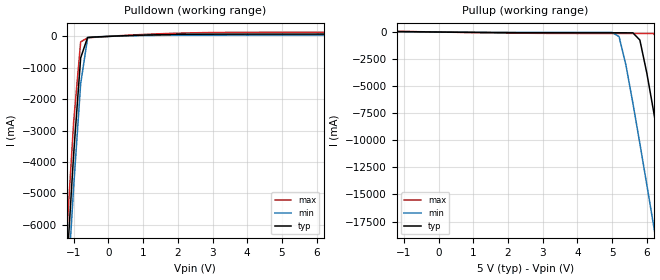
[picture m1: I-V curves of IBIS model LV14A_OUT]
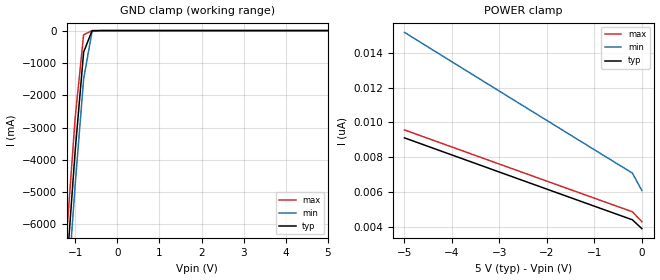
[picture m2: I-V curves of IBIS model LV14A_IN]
|   TEXAS INSTRUMENTS INCORPORATED
|   Advanced Bus Interface Group
|   IBIS Model of LV14A (Vcc=5V)
|   CMOS Hex Schmitt-Trigger Inverter
|   SOIC 14-pin (D) Package
[IBIS Ver]   1.1
[File Name]   lv14a_5.ibs
[File Rev]   2.0
[Date]   9/6/97
[Source]   File originated at Texas Instruments, Inc.
[Notes]   The following is an IBIS list for the LV14A.
|   - All test data contained in this file are derived from
|   hspice(tm) simulations.
|   - File created by Teruo Ishii, SLL Applications.
[Disclaimer] Property of Texas Instruments Incorporated.  Unauthorized
   reproduction and/or distribution is strictly prohibited.
   This product is protected under copyright law.
   Created 1997, (C) Copyright 1997, Texas Instruments Inc.,
   All Rights Reserved
   UNLESS THERE IS A SIGNED, WRITTEN AGREEMENT TO THE
   CONTRARY, TEXAS INSTRUMENTS ("TI") IS PROVIDING THE IBIS
   MODELS "AS IS" AND WITHOUT ANY WARRANTY, EXPRESSED OR
   IMPLIED.  TI assumes no liability for:
   1) the accuracy of the IBIS models provided to your
   company;
   2) the proper functioning of these IBIS models in your
   design or for any resulting applications; or
   3) infringement of patents, copyrights or intellectual
   property rights resulting from your use of these IBIS
   models.
   TI provides IBIS Models as a service to our customers.
   You and your company shall not distribute, sell or give
   these models to anyone else without prior written
   permission from TI.
   TI reserves the right to make changes to our products or
   to discontinue any semiconductor product or service
   without notice, and advises our customers to obtain the
   latest version of relevant information to verify, before
   placing orders, that the information being relied on is
   current.
   Please be aware that your receipt and use of the IBIS
   information provided shall serve as acceptance of these
   terms and conditions.  If you do not accept these terms,
   you should return or destroy the IBIS models and any
   other accompanying information immediately.
[Component]   LV14A(Hex_Inverter)
[Manufacturer]  Texas Instruments
[Package]
|   typ   min   max
R_pkg   0.020   0.018   0.021
L_pkg   3.17nH   2.22nH   4.32nH
C_pkg   0.35pF   0.20pF   0.50pF
[Pin]   signal_name   model_name   R_pin   L_pin   C_pin
1   1A   LV14A_IN   0.018   4.30nH   0.50pF
2   1Y   LV14A_OUT   0.021   3.39nH   0.43pF
3   2A   LV14A_IN   0.019   2.24nH   0.26pF
4   2Y   LV14A_OUT   0.020   2.27nH   0.21pF
5   3A   LV14A_IN   0.020   2.22nH   0.20pF
6   3Y   LV14A_OUT   0.021   3.43nH   0.38pF
7   GND   GND   0.020   4.32nH   0.50pF
8   4Y   LV14A_OUT   0.020   4.32nH   0.50pF
9   4A   LV14A_IN   0.021   3.43nH   0.38pF
10   5Y   LV14A_OUT   0.020   2.22nH   0.20pF
11   5A   LV14A_IN   0.020   2.27nH   0.21pF
12   6Y   LV14A_OUT   0.019   2.24nH   0.26pF
13   6A   LV14A_IN   0.021   3.39nH   0.43pF
14   VCC   POWER   0.018   4.30nH   0.50pF
| Models and submodels in the file (2): LV14A_OUT (Output), LV14A_IN (Input)
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|   Model LV14A_OUT
[Model]   LV14A_OUT
Model_type   Output
Polarity   Inverting
|variable   typ   min   max
C_comp   4.0pF   NA   NA
[Voltage range]   5.0   4.5   5.5
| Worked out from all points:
|   slope of the pulldown table from 0 to 0.75 V, typ, clamps not added: 23.2 ohm
|   slope of the pullup table from 0 to 0.75 V, typ, clamps not added: 29.3 ohm
[Pulldown]
|   Voltage   I(typ)   I(min)   I(max)
-5V       -81.99A    -82.92A    -81.08A
-1.2V     -7.334A    -8.394A    -6.29A
-1V       -3.716A    -4.76A     -2.696A
-800mV    -684.6mA   -1.507A    -174.2mA
-600mV    -32.04mA   -49.56mA   -44.95mA
-400mV    -20.26mA   -14.47mA   -29.3mA
400mV     18.84mA    13.27mA    27.19mA
2.4V      67.49mA    39.34mA    113mA
6.8V      78.71mA    45.01mA    135.4mA
10V       118.3mA    69.61mA    192.4mA
[Pullup]   | Note: Vtable = Vcc - Voutput
|   Voltage   I(typ)   I(min)   I(max)
-5V       52.65mA    31.36mA    86.73mA
5V        -72.3mA    -39.77mA   -130.3mA
5.2V      -72.34mA   -419.6mA   -130.3mA
5.4V      -72.64mA   -3.083A    -130.4mA
5.6V      -75.89mA   -6.59A     -130.4mA
5.8V      -740.7mA   -10.3A     -130.8mA
6.2V      -7.404A    -17.94A    -139.2mA
6.4V      -11.17A    -21.82A    -1.238A
6.8V      -18.88A    -29.62A    -8.294A
7.2V      -26.69A    -37.47A    -15.98A
7.4V      -30.61A    -41.4A     -19.88A
10V       -82.06A    -92.89A    -71.28A
[Ramp]
|Variable   typ   min   max
dV/dt_r   1.7570E+00/2.9778E-09  1.1072E+00/4.7601E-09  2.3491E+00/1.6010E-09
dV/dt_f   1.8625E+00/2.0619E-09  1.1968E+00/3.9150E-09  2.4644E+00/1.1085E-09
|   Model LV14A_IN
[Model]   LV14A_IN
Model_type   Input
Polarity   Inverting
Vinl = 3.5V
Vinh = 1.5V
|variable   typ   min   max
C_comp   2.3pF   NA   NA
[Voltage Range]   5.0   4.5   5.5
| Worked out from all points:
|   GND clamp passes 1 mA (typ) near -0.46 V on its own axis
[GND_Clamp]
|   Voltage   I(typ)   I(min)   I(max)
-5V       -82A       -82.93A    -81.1A
-1.2V     -7.333A    -8.394A    -6.288A
-1V       -3.712A    -4.759A    -2.688A
-800mV    -668.4mA   -1.501A    -130.8mA
-600mV    -3.037mA   -30.13mA   -3.193mA
-400mV    -173.2uA   -104.7uA   -839.2uA
5V        3.916nA    7.599nA    3.537nA
[POWER_Clamp]   | Note: Vtable = Vcc - Voutput
|   Voltage   I(typ)   I(min)   I(max)
-5V       9.116nA    15.16nA    9.57nA
-2.4V     6.569nA    10.78nA    7.027nA
-200mV    4.423nA    7.098nA    4.883nA
0V        3.916nA    6.098nA    4.314nA
